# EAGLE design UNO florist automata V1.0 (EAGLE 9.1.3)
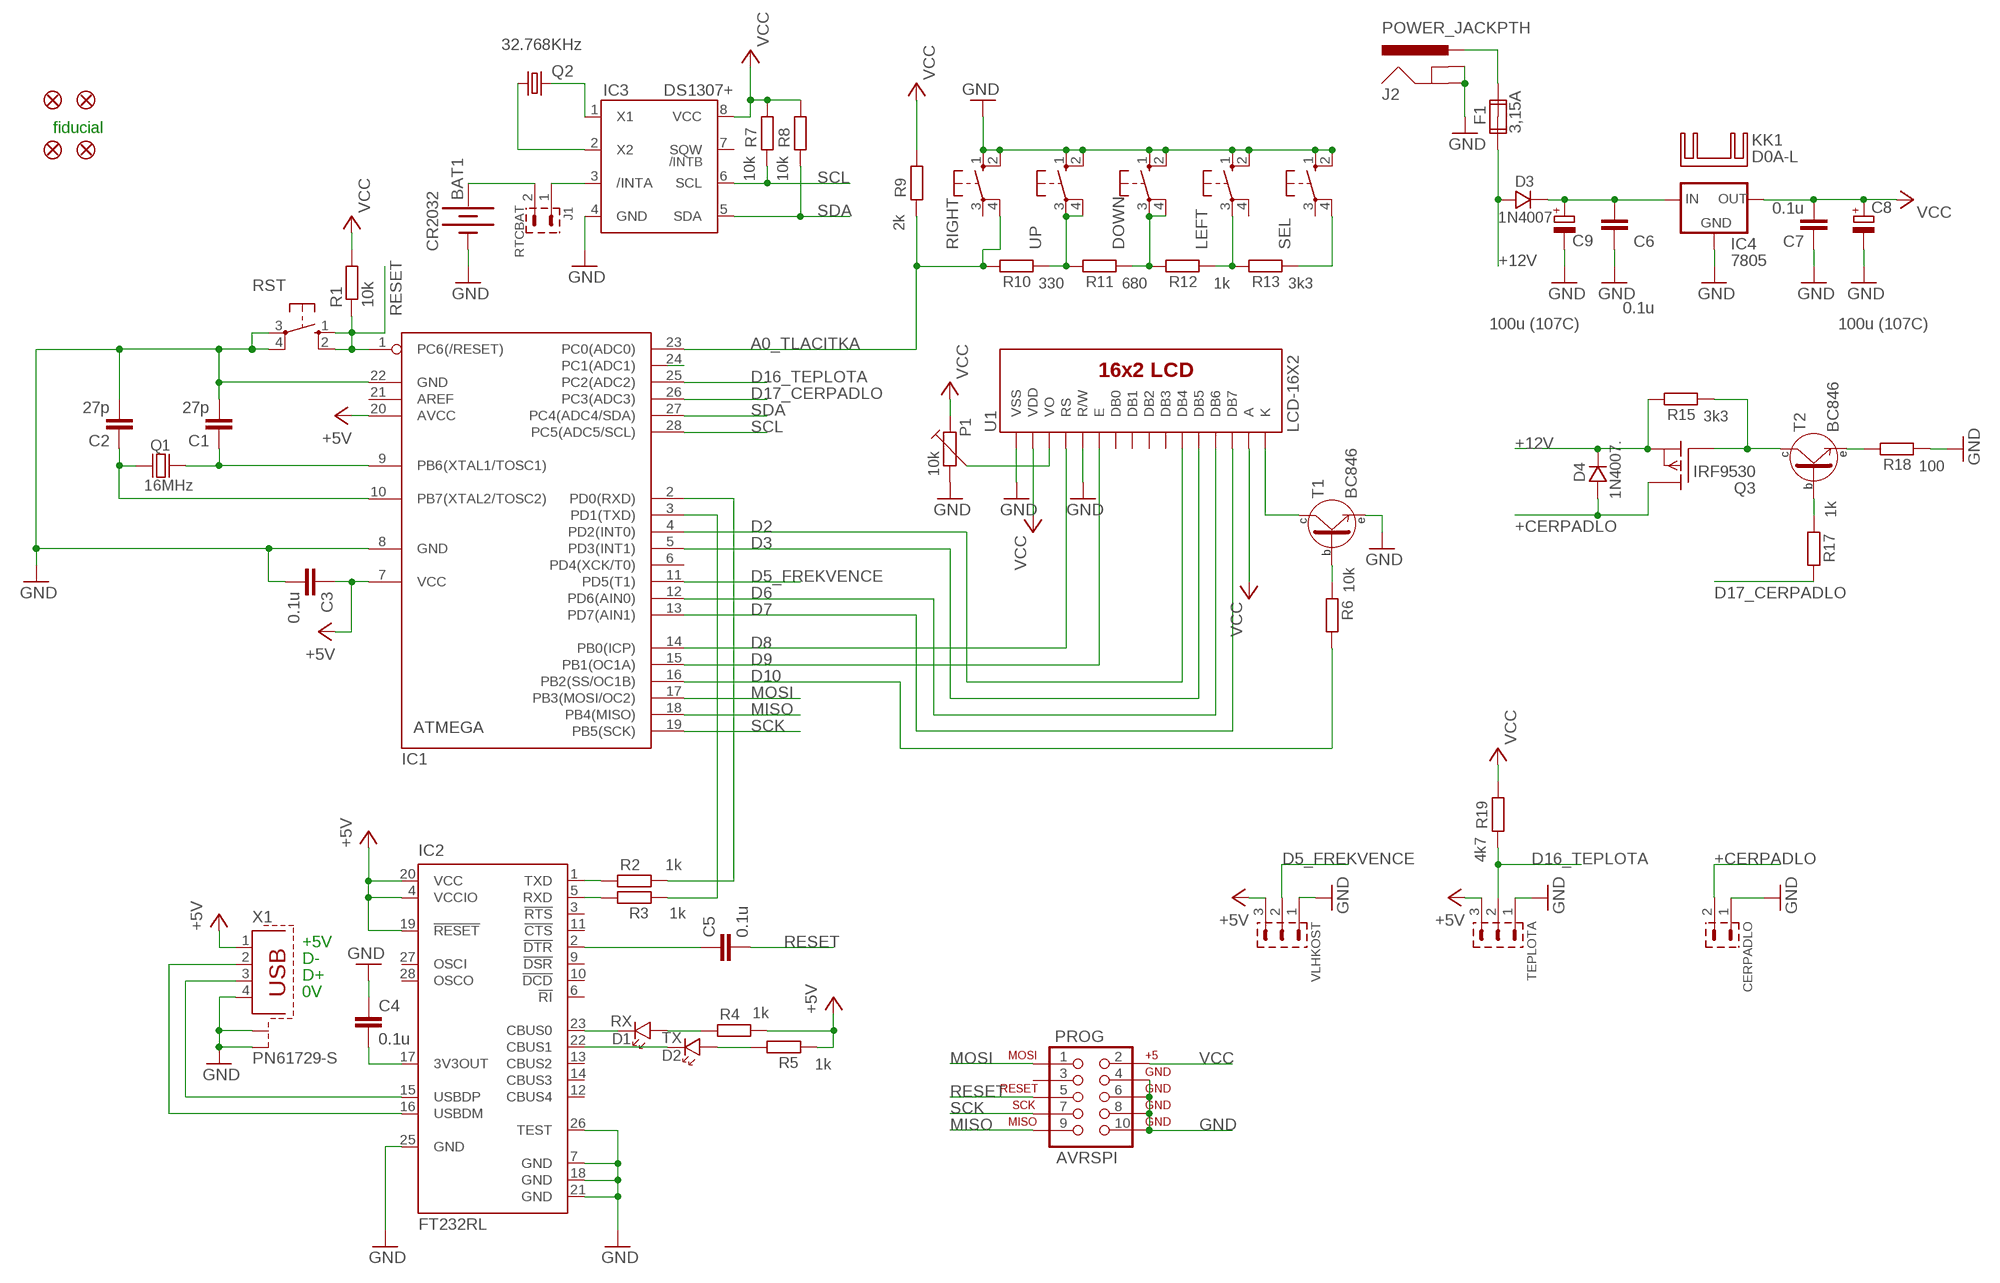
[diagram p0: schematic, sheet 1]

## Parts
BAT1  CR2032  BATTERY20PTH  [BATTCOM_20MM_PTH]
C1  27p  C-EUC1206  [C1206]
C2  27p  C-EUC1206  [C1206]
C3  0.1u  C-EUC1206  [C1206]
C4  0.1u  C-EUC1206  [C1206]
C5  0.1u  C-EUC1206  [C1206]
C6  0.1u  C-EUC1206  [C1206]
C7  0.1u  C-EUC1206  [C1206]
C8  100u (107C)  CPOL-EUC/6032-28W  [C/6032-28W]
C9  100u (107C)  CPOL-EUC/6032-28W  [C/6032-28W]
CERPADLO  PSH02-02P  [PSH02-02P]
D1  RX  LED_1206  [P1206]
D2  TX  LED_1206  [P1206]
D3  1N4007.  [SM-1]
D4  1N4007.  [SM-1]
DOWN  10-XX  [B3F-10XX]
F1  3,15A  FUSE2P  [FUSE1]
FID1  FIDUCIAL1.5X3  [FIDUCIAL-1.5X3]
FID2  FIDUCIAL1.5X3  [FIDUCIAL-1.5X3]
FID3  FIDUCIAL1.5X3  [FIDUCIAL-1.5X3]
FID4  FIDUCIAL1.5X3  [FIDUCIAL-1.5X3]
IC1  ATMEGA  MEGA8-P  [DIL28-3]
IC2  FT232RL  [SSOP28]
IC3  DS1307+  DS1337S+  [SO08]
IC4  7805  78XXL  [78XXL]
J1  RTCBAT  S1G2_JUMP  [S1G2_JUM]
J2  POWER_JACKPTH  [POWER_JACK_PTH]
KK1  D0A-L  [D02A-L]
LEFT  10-XX  [B3F-10XX]
P1  10k  TRIMRPT10V  [PT10V]
PROG  AVRSPI  AVR_SPI_PROG2LOCK  [2X5-SHROUDED_LOCK]
Q1  16MHz  Q_HC-49U  [HC-49U]
Q2  32.768KHz  CRYSTALTC38H  [TC38H]
Q3  IRF9530  [TO220]
R1  10k  R-EU_M1206  [M1206]
R2  1k  R-EU_M1206  [M1206]
R3  1k  R-EU_M1206  [M1206]
R4  1k  R-EU_M1206  [M1206]
R5  1k  R-EU_M1206  [M1206]
R6  10k  R-EU_M1206  [M1206]
R7  10k  R-EU_M1206  [M1206]
R8  10k  R-EU_M1206  [M1206]
R9  2k  R-EU_M1206  [M1206]
R10  330  R-EU_M1206  [M1206]
R11  680  R-EU_M1206  [M1206]
R12  1k  R-EU_M1206  [M1206]
R13  3k3  R-EU_M1206  [M1206]
R15  3k3  R-EU_M1206  [M1206]
R17  1k  R-EU_M1206  [M1206]
R18  100  R-EU_M1206  [M1206]
R19  4k7  R-EU_M1206  [M1206]
RIGHT  10-XX  [B3F-10XX]
RST  10-XX  [B3F-10XX]
SEL  10-XX  [B3F-10XX]
T1  BC846  [SOT-23]
T2  BC846  [SOT-23]
TEPLOTA  PSH02-03P  [PSH02-03P]
U1  LCD-16X2  LCD-16X2NOSILK  [LCD-16X2_NOSILK]
UP  10-XX  [B3F-10XX]
VLHKOST  PSH02-03P  [PSH02-03P]
X1  PN61729-S  [PN61729-S]

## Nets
+12V: D3.A D4.K F1.1A Q3.3(S) R15.2
+CERPADLO: CERPADLO.2 D4.A Q3.2(D)
A: IC3.2(X2) Q2.1
A0_TLACITKA: IC1.23(PC0(ADC0)) R9.1 R10.2 RIGHT.4(P1)
A1_OSVETLENI: IC1.24(PC1(ADC1))
D2: IC1.4(PD2(INT0)) U1.11(DB4)
D3: IC1.5(PD3(INT1)) U1.12(DB5)
D5_FREKVENCE: IC1.11(PD5(T1)) VLHKOST.2
D6: IC1.12(PD6(AIN0)) U1.13(DB6)
D7: IC1.13(PD7(AIN1)) U1.14(DB7)
D8: IC1.14(PB0(ICP)) U1.4(RS)
D9: IC1.15(PB1(OC1A)) U1.6(E)
D10: IC1.16(PB2(SS/OC1B)) R6.2
D16_TEPLOTA: IC1.25(PC2(ADC2)) R19.1 TEPLOTA.2
D17_CERPADLO: IC1.26(PC3(ADC3)) R17.2
GND: BAT1.2(-) C1.2 C2.2 C3.2 C4.1 C6.1 C7.1 C8.- C9.- CERPADLO.1 DOWN.1(S) DOWN.2(S1) IC1.8(GND) IC1.22(GND) IC2.7(GND) IC2.18(GND) IC2.21(GND) IC2.25(GND) IC2.26(TEST) IC3.4(GND) IC4.GND J2.GND J2.GNDBREAK LEFT.1(S) LEFT.2(S1) P1.2 PROG.4 PROG.6 PROG.8 PROG.10 R18.1 RIGHT.1(S) RIGHT.2(S1) RST.3(P) RST.4(P1) SEL.1(S) SEL.2(S1) T1.2(E) TEPLOTA.1 U1.1(VSS) U1.5(R/W) UP.1(S) UP.2(S1) VLHKOST.1 X1.4 X1.S1 X1.S2
MISO: IC1.18(PB4(MISO)) PROG.9
MOSI: IC1.17(PB3(MOSI/OC2)) PROG.1
N$1: IC2.16(USBDM) X1.2
N$2: IC2.15(USBDP) X1.3
N$3: C4.2 IC2.17(3V3OUT)
N$4: IC2.1(TXD) R2.1
N$5: IC2.5(RXD) R3.2
N$6: IC1.2(PD0(RXD)) R2.2
N$7: IC1.3(PD1(TXD)) R3.1
N$8: C5.1 IC2.2(!DTR)
N$9: D1.K IC2.23(CBUS0)
N$10: D1.A R4.1
N$11: D2.K IC2.22(CBUS1)
N$12: D2.A R5.2
N$13: BAT1.1(+) J1.2
N$14: IC3.3(/INTA) J1.1
N$15: T1.3(C) U1.16(K)
N$18: R10.1 R11.2 UP.3(P) UP.4(P1)
N$19: DOWN.3(P) DOWN.4(P1) R11.1 R12.2
N$20: LEFT.3(P) R12.1 R13.2
N$21: R13.1 SEL.4(P1)
N$22: F1.2A J2.PWR
N$23: C1.1 IC1.9(PB6(XTAL1/TOSC1)) Q1.2
N$24: C6.2 C9.+ D3.K IC4.IN
N$25: R6.1 T1.1(B)
N$26: C2.1 IC1.10(PB7(XTAL2/TOSC2)) Q1.1
N$27: Q3.1(G) R15.1 T2.3(C)
N$28: R18.2 T2.2(E)
N$29: R17.1 T2.1(B)
N$31: P1.3 U1.3(VO)
Q1: IC3.1(X1) Q2.2
RESET: C5.2 IC1.1(PC6(/RESET)) PROG.5 R1.1 RST.1(S) RST.2(S1)
SCK: IC1.19(PB5(SCK)) PROG.7
SCL: IC1.28(PC5(ADC5/SCL)) IC3.6(SCL) R7.1
SDA: IC1.27(PC4(ADC4/SDA)) IC3.5(SDA) R8.1
VCC: C3.1 C7.2 C8.+ IC1.7(VCC) IC1.20(AVCC) IC2.4(VCCIO) IC2.19(!RESET) IC2.20(VCC) IC3.8(VCC) IC4.OUT P1.1 PROG.2 R1.2 R4.2 R5.1 R7.2 R8.2 R9.2 R19.2 TEPLOTA.3 U1.2(VDD) U1.15(A) VLHKOST.3 X1.1 ; supply symbol labelled +5V
Unconnected: F1.1B F1.2B IC1.6(PD4(XCK/T0)) IC1.21(AREF) IC2.3(!RTS) IC2.6(!RI) IC2.9(!DSR) IC2.10(!DCD) IC2.11(!CTS) IC2.12(CBUS4) IC2.13(CBUS2) IC2.14(CBUS3) IC2.27(OSCI) IC2.28(OSCO) IC3.7(SQW) LEFT.4(P1) PROG.3 RIGHT.3(P) SEL.3(P) U1.7(DB0) U1.8(DB1) U1.9(DB2) U1.10(DB3)

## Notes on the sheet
- fiducial
- +5V
- D-
- D+
- 0V

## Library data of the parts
BAT1 = SparkFun-Electromechanical:BATTERY: Battery Holders
C1-C7 = rcl:C-EU: CAPACITOR, European symbol
C8 C9 = rcl:CPOL-EU: POLARIZED CAPACITOR, European symbol
CERPADLO = #PaJa_konektory:PSH02-02: Konektory se zamkem - vidlice - 2pin
D1 D2 = #PaJa_31:LED: LED - jednobarevna
D3 D4 = #PaJa_31:1N4007: Usmernovaci dioda - 1A, 1000V
DOWN LEFT RIGHT RST SEL UP = switch-omron-modified:10-XX: OMRON SWITCH
F1 = special:FUSE2P: FUSE 5 x 20 mm
FID1-FID4 = SparkFun-Retired:FIDUCIAL: Fiducial Alignment Points
IC1 = atmel:MEGA8-P: MICROCONTROLLER 8 Kbytes FLASH, 1 kbytes SRAM, 512 bytes EEPROM, USART, 4-channel 10 bit ADC, 2-channel 8 bit ADC Pin compatible with Atmega48, ATMega88, ATMega168 Source: avr.lbr
IC2 = ftdichip:FT232R: Source: http://www.ftdichip.com/Documents/DataSheets/DS_FT232R_v104.pdf; MPN: FT232RL; OC_FARNELL: 1146032; OC_NEWARK: 91K9918
IC3 = #PaJa_31:DS1337: RTC - obvod realneho casu (ekviv. DS1307)
IC4 = v-reg:78XXL: VOLTAGE REGULATOR
J1 = #PaJa_konektory:S1G2_JUMP: Radove konektory - koliky - 2x
J2 = SparkFun-Connectors:POWER_JACK: Power Jack This is the standard 5.5mm barrel jack for power. The PTH is the most common, proven, reliable, footprint. The Slot footprint only works if the mill layer is transmitted to the PCB fab house so be warned. Mating wall wart : TOL-00298 (and others); PROD_ID: PRT-00119
KK1 = heatsink:D0A-L: HEATSINK
P1 = #PaJa_31:TRIMR: Trimr
PROG = SparkFun-Connectors:AVR_SPI_PROG2: AVR 10-pin ICSP Header This is the standard AVR In Circuit Serial Programming header. Minimal, but includes pin one indicator. Works with standard Olimex programmers. Also look for the 6-pin reduced version. Spark Fun Electronics SKU: PRT-00778
Q1 = #PaJa_31:Q: Krystal
Q2 = crystal:CRYSTAL: CRYSTAL; OC_FARNELL: unknown; OC_NEWARK: unknown
Q3 = transistor-fet:IRF9530: P-Channel Enhancement MOSFET (HEXFET); -100V; -12A; 0,3Ohm
R1-R13 R15 R17-R19 = rcl:R-EU_: RESISTOR, European symbol
T1 T2 = #PaJa_31:BC846: SMD tranzistor - NPN - ekv. BC546
TEPLOTA VLHKOST = #PaJa_konektory:PSH02-03: Konektory se zamkem - vidlice - 3pin
U1 = SparkFun-Displays:LCD-16X2: Standard text-only 16x2 parallel input LCD
X1 = con-berg:PN61729-S: BERG USB connector; OC_FARNELL: unknown; OC_NEWARK: unknown

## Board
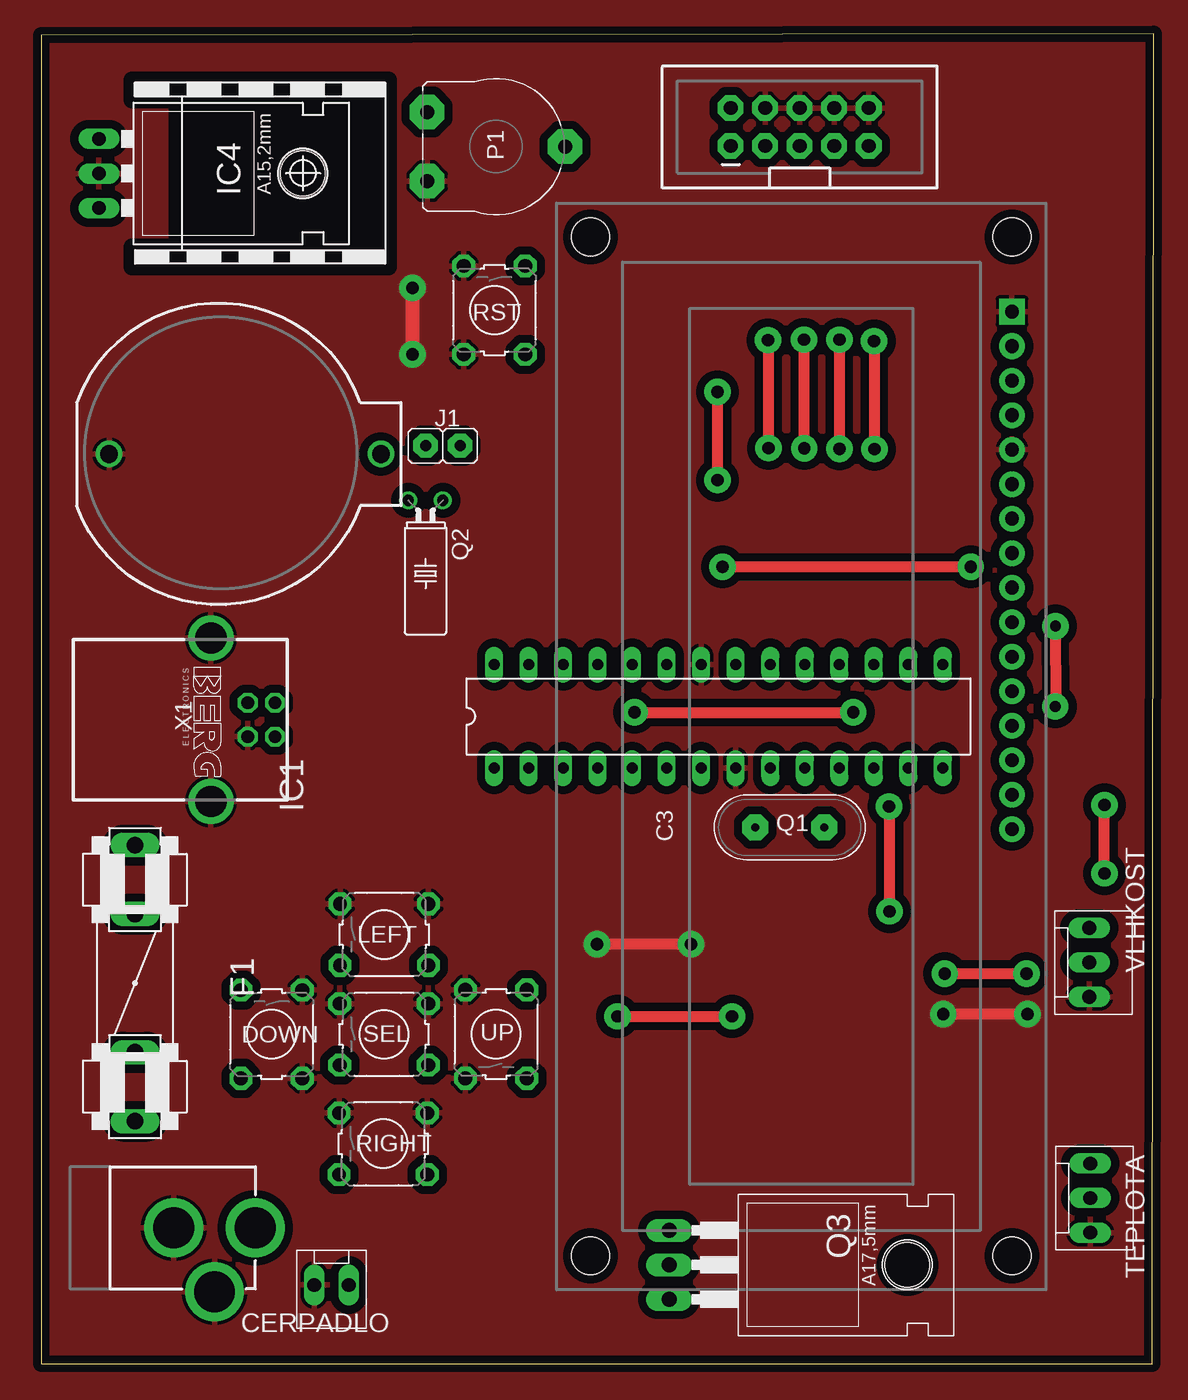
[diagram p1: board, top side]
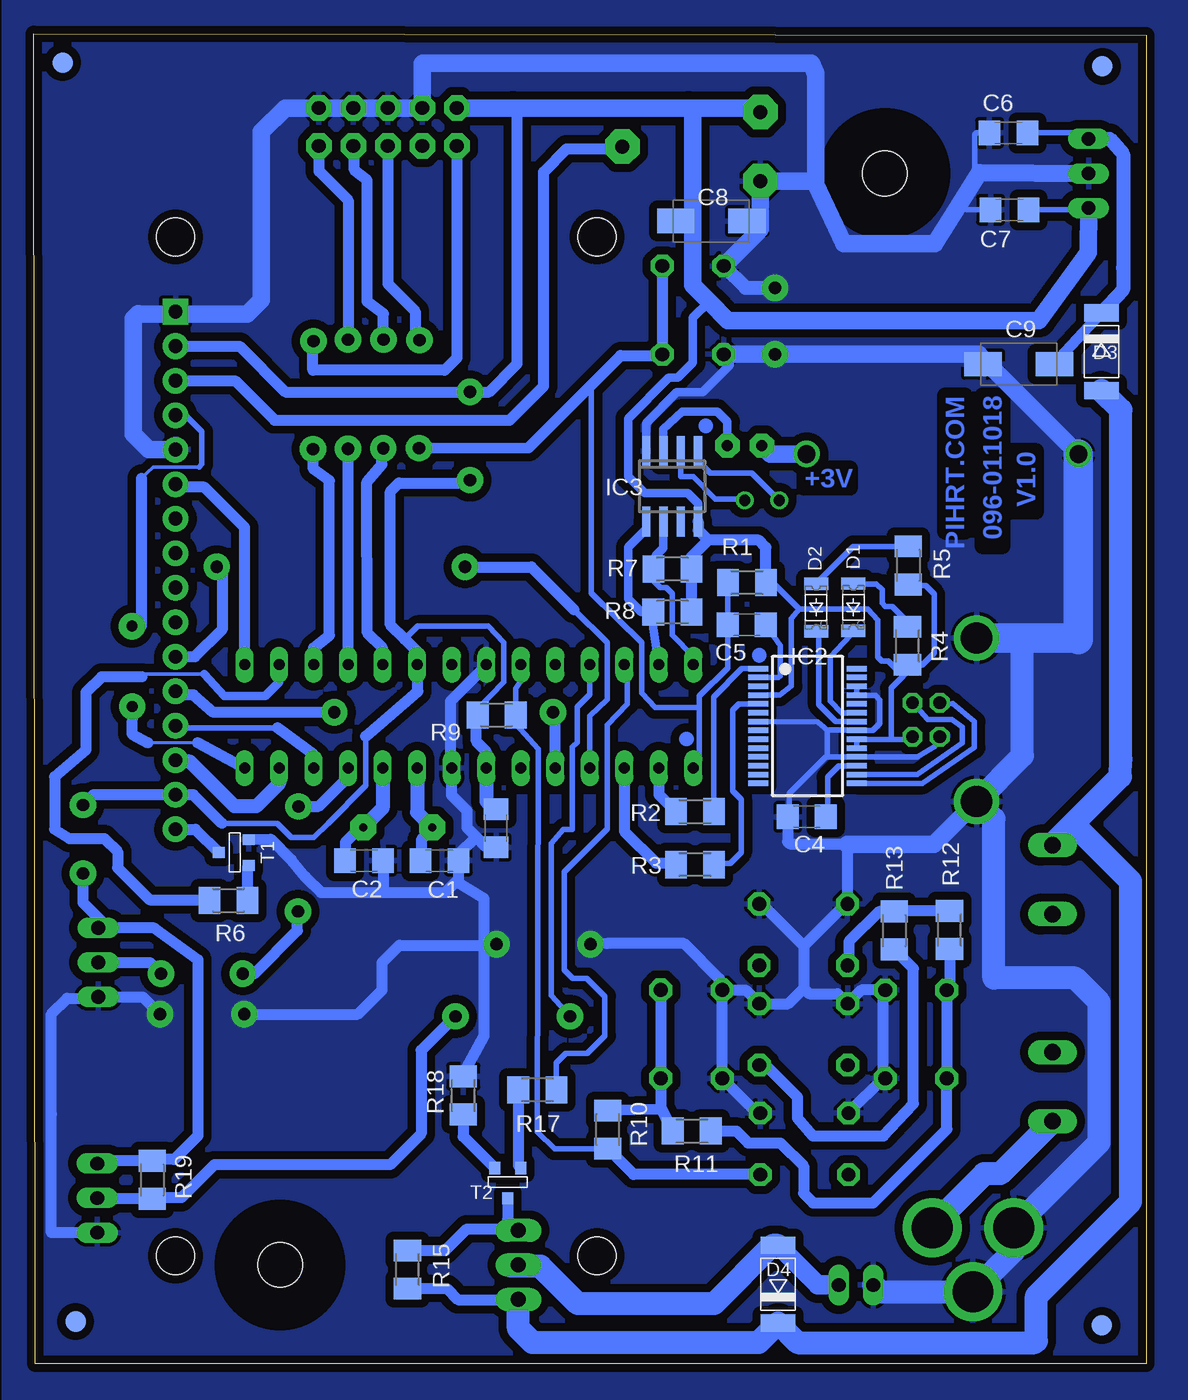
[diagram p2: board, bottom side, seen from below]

Size 81.85 x 97.9 mm. Coordinates in mm from the lower left corner, seen from the top.
Outline: 0.02,0.01 81.76,0 81.85,97.9 0,97.8 0.02,0.01
Copper layers (1*16): Top 0.035mm / dielectric 1.5mm / Bottom 0.035mm
Design rules "default": minimum track width 5mil, minimum drill 12mil, track to track 5mil, track to pad 5mil, pad to pad 5mil, via to via 5mil, smd to smd 0mil, copper to edge 10mil, drill to drill 10mil, minimum pad ring 10mil, minimum via ring 6mil, stop-mask expansion 2mil, vias tented up to drill 25mil, thermal gap 10mil

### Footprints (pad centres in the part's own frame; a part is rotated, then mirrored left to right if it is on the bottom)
BATTCOM_20MM_PTH = drill 1.3: 1 11.85,0; 2 -8.15,0
C1206 = smd 1.6 x 1.8: 1 -1.4,0; 2 1.4,0
C/6032-28W = smd 2.75 x 1.8: + 2.625,0; - -2.625,0
PSH02-02P = drill 1.016 pad 1.422 long: 1 -1.27,0; 2 1.27,0
P1206 = smd 0.914 x 1.778: A -1.905,0; K 1.587,0
SM-1 = smd 1.27 x 2.54: A 2.857,0; K -2.857,0
B3F-10XX = drill 1.016 pad 1.676 octagon: 1 -3.251,2.261; 2 3.251,2.261; 3 -3.251,-2.261; 4 3.251,-2.261
FUSE1 = drill 1.194 long: 1A -10.16,0; 1B -5.08,0; 2A 10.16,0; 2B 5.08,0
FIDUCIAL-1.5X3 = smd 1.5 x 1.5: 1 0,0
DIL28-3 = drill 0.813 long: 1 -16.51,-3.81; 2 -13.97,-3.81; 3 -11.43,-3.81; 4 -8.89,-3.81; 5 -6.35,-3.81; 6 -3.81,-3.81; 7 -1.27,-3.81; 8 1.27,-3.81; 9 3.81,-3.81; 10 6.35,-3.81; 11 8.89,-3.81; 12 11.43,-3.81; 13 13.97,-3.81; 14 16.51,-3.81; 15 16.51,3.81; 16 13.97,3.81; 17 11.43,3.81; 18 8.89,3.81; 19 6.35,3.81; 20 3.81,3.81; 21 1.27,3.81; 22 -1.27,3.81; 23 -3.81,3.81; 24 -6.35,3.81; 25 -8.89,3.81; 26 -11.43,3.81; 27 -13.97,3.81; 28 -16.51,3.81
SSOP28 = smd 0.4 x 1.5: 1 -4.225,-3.625; 2 -3.575,-3.625; 3 -2.925,-3.625; 4 -2.275,-3.625; 5 -1.625,-3.625; 6 -0.975,-3.625; 7 -0.325,-3.625; 8 0.325,-3.625; 9 0.975,-3.625; 10 1.625,-3.625; 11 2.275,-3.625; 12 2.925,-3.625; 13 3.575,-3.625; 14 4.225,-3.625; 15 4.225,3.625; 16 3.575,3.625; 17 2.925,3.625; 18 2.275,3.625; 19 1.625,3.625; 20 0.975,3.625; 21 0.325,3.625; 22 -0.325,3.625; 23 -0.975,3.625; 24 -1.625,3.625; 25 -2.275,3.625; 26 -2.925,3.625; 27 -3.575,3.625; 28 -4.225,3.625
SO08 = smd 0.6 x 2.2: 1 -1.905,-2.6; 2 -0.635,-2.6; 3 0.635,-2.6; 4 1.905,-2.6; 5 1.905,2.6; 6 0.635,2.6; 7 -0.635,2.6; 8 -1.905,2.6
78XXL = drill 1.016 long: GND 0,-3.81; IN -2.54,-3.81; OUT 2.54,-3.81 | hole 3.302: 0,11.176
S1G2_JUM = drill 0.813 pad 1.778 octagon: 1 -1.27,0; 2 1.27,0
POWER_JACK_PTH = drill 2.997 pad 4.318: GND 0,7.7; GNDBREAK 4.7,10.7; PWR 0,13.7
PT10V = drill 1.016 pad 2.54 octagon: 1 -2.54,-5.08; 2 2.54,-5.08; 3 0,5.08
2X5-SHROUDED_LOCK = drill 1.016 pad 1.88 octagon: 1 -1.397,5.08; 2 1.397,5.08; 3 -1.397,2.54; 4 1.397,2.54; 5 -1.397,0; 6 1.397,0; 7 -1.397,-2.54; 8 1.397,-2.54; 9 -1.397,-5.08; 10 1.397,-5.08
HC-49U = drill 0.61 pad 1.93 octagon: 1 -2.54,0; 2 2.54,0
TC38H = drill 0.813: 1 -1.27,0; 2 1.27,0
TO220 = drill 1.118 long: 1 -2.54,-6.35; 2 0,-6.35; 3 2.54,-6.35 | hole 3.302: 0,11.176
M1206 = smd 1.6 x 2: 1 -1.4,0; 2 1.4,0
SOT-23 = smd 0.787 x 0.889: 1 -0.953,-0.953; 2 0.953,-0.953; 3 0,1.27
PSH02-03P = drill 1.016 pad 1.422 long: 1 -2.54,0; 2 0,0; 3 2.54,0
LCD-16X2_NOSILK = drill 1.016 pad 1.88 square: 1 -32,15.5 | drill 1.016 pad 1.88: 2 -29.46,15.5; 3 -26.92,15.5; 4 -24.38,15.5; 5 -21.84,15.5; 6 -19.3,15.5; 7 -16.76,15.5; 8 -14.22,15.5; 9 -11.68,15.5; 10 -9.14,15.5; 11 -6.6,15.5; 12 -4.06,15.5; 13 -1.52,15.5; 14 1.02,15.5; 15 3.56,15.5; 16 6.1,15.5 | hole 2.8: -37.5,15.5; -37.5,-15.5; 37.5,15.5; 37.5,-15.5
PN61729-S = drill 0.95 octagon: 1 1.25,4.71; 2 -1.25,4.71; 3 -1.25,2.71; 4 1.25,2.71 | drill 2.3 pad 2.9: S1 -6.02,0; S2 6.02,0

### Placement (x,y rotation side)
BAT1  13.16,66.97 0 top
C1  52.02,37.05 0 bottom
C2  57.57,37.05 0 bottom
C3  47.86,39.43 270 bottom
C4  25,40.27 0 bottom
C5  29.41,54.41 180 bottom
C6  10.15,90.61 0 bottom
C7  10.07,84.95 0 bottom
C8  32.01,84.13 180 bottom
C9  9.4,73.59 0 bottom
CERPADLO  21.37,5.81 0 top
D1  21.56,55.54 270 bottom
D2  24.3,55.53 270 bottom
D3  3.3,74.51 270 bottom
D4  27.09,5.87 90 bottom
DOWN  16.96,24.27 270 top
F1  6.9,28.03 270 top
FID1  3.24,95.51 0 bottom
FID2  3.28,2.84 0 bottom
FID3  79.75,95.8 0 bottom
FID4  78.79,3.12 0 bottom
IC1  49.84,47.67 0 top
IC2  24.94,46.96 270 bottom
IC3  34.9,64.61 180 bottom
IC4  8.07,87.63 270 top
J1  29.56,67.59 180 top
J2  2.06,10.02 270 top
KK1  13.81,87.64 180 top
LEFT  25.25,31.61 0 top
P1  33.48,89.6 270 top
PROG  55.82,91.05 90 top
Q1  55.08,39.5 180 top
Q2  28.29,63.57 180 top
Q3  52.56,7.3 270 top
R1  29.39,57.51 0 bottom
R2  33.22,40.66 180 bottom
R3  33.22,36.74 0 bottom
R4  17.58,52.86 270 bottom
R5  17.52,58.78 90 bottom
R6  67.54,34.13 180 bottom
R7  34.87,58.52 0 bottom
R8  34.88,55.34 0 bottom
R9  47.81,47.76 180 bottom
R10  39.63,17.26 270 bottom
R11  33.45,17.15 180 bottom
R12  14.49,31.94 270 bottom
R13  18.55,31.91 90 bottom
R15  54.37,6.95 270 bottom
R17  44.81,20.18 0 bottom
R18  50.27,19.77 270 bottom
R19  73.15,13.55 90 bottom
RIGHT  25.17,16.21 0 top
RST  33.36,77.57 270 top
SEL  25.23,24.26 0 top
T1  66.99,37.65 90 bottom
T2  46.99,13.47 180 bottom
TEPLOTA  77.19,12.21 90 top
U1  55.94,45.46 270 top
UP  33.48,24.28 90 top
VLHKOST  77.13,29.55 90 top
X1  12.5,47.42 270 top

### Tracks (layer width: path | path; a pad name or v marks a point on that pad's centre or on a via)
+12V
  Bottom 0.813: R15.2 51.48,5.55 50.65,4.73 46.24,4.73 Q3.3
  Bottom 1.676: D3.A 1.88,70.23 1.88,44.51 1.92,43.24 5.56,39.6 | 5.56,39.6 6.9,38.26 F1.1A | Q3.3 46.21,2.61 45.15,1.56 28.55,1.56 D4.K 25.64,1.56 8.23,1.56 8.09,1.69 8.09,5 1.15,11.94 1.15,35.52 5.23,39.6 5.56,39.6
+CERPADLO
  Bottom 1.422: CERPADLO.2 24.18,5.81 D4.A
  Bottom 1.676: D4.A 27.52,8.73 31.81,4.44 41.84,4.44 44.59,7.2 46.75,7.2 46.8,7.25 46.25,7.25 Q3.2
A
  Bottom 0.406: Q2.1 29.66,63.67 31.72,63.67 33.35,65.3 34.27,65.3 IC3.2
A0_TLACITKA
  Bottom 0.406: IC1.23 45.84,51.29 45.84,50.53 46.41,49.7 R9.1 46.41,47.12 44.77,45.26 44.81,17.1 43.54,15.83 39.66,15.83 R10.2
  Bottom 0.813: R10.2 37.72,13.94 RIGHT.4
D2  (via drill 0.9 pad 1.93)
  Top 0.813: v68.4,58.67 v50.14,58.67
  Bottom 0.406: IC1.4 40.95,47.68 39.67,48.92 39.67,53.12 42.12,55.53
  Bottom 0.813: U1.11 70.02,52.06 67.97,54.1 67.97,58.24 v68.4,58.67 | v50.14,58.67 45.26,58.67 42.12,55.53
D3  (via drill 0.9 pad 1.93)
  Top 0.813: v43.66,47.97 v59.76,47.97
  Bottom 0.813: IC1.5 43.49,47.64 v43.66,47.97 | v59.76,47.97 68.65,47.97 70.12,49.25 71.17,49.25 U1.12
D5_FREKVENCE  (via drill 0.9 pad 1.93)
  Top 0.813: v72.5,28.73 v66.5,28.73 | v62.43,33.31 62.43,41 v62.39,41.04
  Bottom 0.813: VLHKOST.2 73.33,29.55 v72.5,28.73 | v66.5,28.73 65.64,28.73 62.47,31.9 62.47,33.28 v62.43,33.31 | v62.39,41.04 60.9,41.04 58.89,43.05 58.89,43.7 IC1.11
D6
  Bottom 0.406: IC1.12 61.27,44.85 | 63.92,46.83 71.04,46.83 U1.13
  Bottom 0.813: 61.27,44.85 63.92,46.83
D7
  Bottom 1.016: IC1.13 63.81,42.74 65.5,41.05 67.09,41.05 70.37,44.34 71.34,44.34 U1.14
D8  (via drill 0.8 pad 1.93)
  Top 0.813: v74.64,54.3 74.65,48.55 v74.63,48.39
  Bottom 0.254: 69.67,66.03 73.09,66.03 73.95,65.19 | 73.45,45.71 69.82,45.73
  Bottom 0.406: U1.4 70.71,69.84 69.5,68.63 69.5,66.23 69.67,66.03
  Bottom 0.813: 73.95,65.19 73.95,54.34 v74.64,54.3 | v74.63,48.39 74.64,46.37 73.45,45.71 | 69.82,45.73 IC1.14
D9
  Bottom 0.813: IC1.15 66.35,61.58 69.31,64.54 71.22,64.54 U1.6
D10
  Bottom 0.254: 69.31,50.8 73.92,50.8 73.9,50.58
  Bottom 0.61: IC1.16 63.81,50.19 64.84,49.16 67.84,49.16 69.31,50.8
  Bottom 0.813: 73.9,50.58 76.88,50.58 78.03,49.43 78.03,45.2 80.33,43.24 80.33,39.36 79.24,38.67 76.66,38.67 75.7,37.71 75.7,36.53 73.34,34.17 68.97,34.17 R6.2
D16_TEPLOTA  (via drill 0.9 pad 1.93)
  Top 0.813: v42.41,25.59 v50.83,25.59
  Bottom 0.406: IC1.25 40.95,49.26 41.86,48.35 41.86,45.76 42.23,45.41 42.23,39.35 42.89,39.35 43.81,38.31 43.81,27.12 v42.41,25.59
  Bottom 0.813: TEPLOTA.2 77.13,12.15 R19.1 73.06,12.24 71.01,12.24 68.59,14.66 55.64,14.66 53.37,16.94 53.37,23.09 50.87,25.59 v50.83,25.59
D17_CERPADLO
  Bottom 0.406: IC1.26 38.19,51.26 38.19,48.57 39.68,47.02 39.68,39.37 42.84,36.21 42.84,29.02 42.22,28.39 41.18,28.39 39.85,27.06 39.85,24.17 41.14,22.88 42.71,22.88 43.41,22.17 R17.2
GND  (via drill 0.9 pad 1.93)
  Top 0.813: v40.91,30.9 v47.82,30.9 | v72.58,25.74 v66.39,25.74
  Top 1.016: v27.32,79.21 v27.32,74.32
  Bottom 0.406: IC2.26 IC2.25 21.27,49.21 19.92,49.21 19.62,48.88 19.62,47.13 20.12,46.64 IC2.21 21.33,46.65 | X1.4 15.58,45.44 16.85,44.67 20.99,44.67 IC2.18 23.58,44.68 | IC2.7 24.18,47.27 23.45,46.63 21.33,46.65 | 23.58,44.68 26.28,41.98 26.28,40.24 26.28,40.07 26.4,40.07 | 21.33,46.65 23.46,46.65 23.5,46.61 23.5,44.77 23.58,44.68 | C6.1 12.5,90.61 12.64,90.47 12.64,88.04 12.29,87.69 | C7.1 13.2,84.95 13.7,85.44
  Bottom 0.61: IC3.4 36.8,69.27 34.54,71.53 32.65,71.53 30.65,73.53 30.65,73.87 RST.4
  Bottom 0.813: C3.2 48.56,38.03 49.33,38.8 | 49.33,38.8 49.98,39.45 49.98,40.72 51.12,41.86 IC1.8 51.21,43.95 51.21,48.77 48.57,51.4 IC1.22 | 49.33,38.8 50.62,37.51 C1.2 50.6,37.03 50.6,35.68 50.77,35.51 | C4.1 26.31,40.27 26.28,40.24 | 26.4,40.07 26.4,38.43 26.26,38.28 22.07,38.28 22.03,38.25 22.03,33.9 LEFT.1 22.14,33.87 25.23,30.78 | T1.2 64.43,38.63 62.91,37.11 61.89,35.86 60.73,34.7 56.04,34.7 | 56.04,34.7 51.58,34.7 50.77,35.51 | C2.2 56.17,34.83 56.04,34.7 | DOWN.2 19.37,21.02 | 19.37,21.02 RIGHT.1 | RIGHT.2 28.66,18.47 UP.1 | 25.23,30.78 25.23,27.66 | 25.23,27.66 24.82,27.25 22.71,27.25 SEL.1 20.97,27.52 DOWN.1 19.37,27.37 19.37,21.02 | 25.23,27.66 26.36,26.52 SEL.2 29.49,27.53 UP.2 UP.1 | LEFT.2 28.31,33.87 25.23,30.78 | 71.63,77.26 U1.1 | UP.1 31.22,27.57 31.41,27.76 31.41,28.35 34.01,30.94 39.7,30.94 v40.91,30.9 | R18.1 50.27,21.3 48.73,24.14 48.73,30.67 | 48.73,30.67 48.73,30.86 | 48.73,30.86 v47.82,30.9 | 48.73,30.86 48.73,34.25 50.77,35.51 | TEPLOTA.1 80.57,9.67 80.58,9.67 80.58,18.41 80.58,25.75 79.41,26.91 77.22,26.91 VLHKOST.1 73.84,27.01 v72.58,25.74 | v66.39,25.74 58.03,25.74 56.24,27.53 56.24,29.55 54.97,30.81 48.88,30.81 48.73,30.67 | C9.- 12.21,74.18 | C8.- 28.68,83.24
  Bottom 1.016: RST.3 29.48,79.21 v27.32,79.21
  Bottom 1.27: RST.3 28.68,83.24 28.4,83.51 P1.2 28.39,87.08 24.6,87.06 | IC4.GND 12.29,87.69 13.7,85.44 15.55,82.47 22.25,82.47 24.36,86.89 24.6,87.06 | 24.6,87.06 24.32,87.13 24.32,94.98 24.67,95.74 53.26,95.74 53.28,95.72 PROG.4 PROG.6 PROG.8 PROG.10 63.37,92.45 65.12,90.7 65.12,78.3 66.15,77.26 71.63,77.26 74.13,77.26 74.17,77.3 74.54,76.92 74.54,68.43 73.41,67.3 U1.5 | RST.4 v27.32,74.32 12.35,74.32 12.21,74.18 BAT1.2 | X1.S2 15.65,38.25 22.03,38.25
  Bottom 1.676: CERPADLO.1 19.6,5.31 J2.GNDBREAK 9.76,8.31 J2.GND 3.47,16.3 3.47,26.63 5.25,28.41 11.22,28.41 11.22,40.12 X1.S2 9.13,44.77 9.13,53.44
  Bottom 2.184: BAT1.2 5.01,53.31 5.14,53.44 9.13,53.44 X1.S1
  pour Bottom (isolate 0.61): -4.02,100.89 -4.02,-2.8 84.05,-2.8 84.05,100.89
  pour Top (isolate 0.61): -4.28,101.93 -4.28,-3.54 85.41,-3.54 85.41,101.93
MISO  (via drill 0.9 pad 1.93)
  Top 0.813: v58.74,75.39 v58.74,67.36
  Bottom 0.813: PROG.9 60.86,89.62 60.86,87.78 58.74,85.66 v58.74,75.39 | IC1.18 v58.73,67.35 v58.74,67.36
MOSI  (via drill 0.9 pad 1.93)
  Top 0.813: v61.29,75.29 61.29,67.38 v61.32,67.35
  Bottom 0.813: IC1.17 61.27,52.7 60.12,53.63 60.12,65.01 61.3,65.89 v61.32,67.35 | PROG.1 50.74,74.04 51.64,73.14 61.32,73.14 61.32,74.92 61.31,74.93 61.31,75.27 v61.29,75.29
N$1
  Bottom 0.406: IC2.16 16.85,43.38 13.55,45.7 13.54,46.88 14.34,47.42 16.09,47.43 X1.2
N$2
  Bottom 0.406: IC2.15 16.48,42.73 12.66,45.36 12.66,47.28 14.24,48.63 15.16,48.59 X1.3
N$3
  Bottom 0.406: IC2.17 22.64,44.03 23.46,43.2 23.46,40.34 23.54,40.2
  Bottom 0.813: C4.2 23.54,40.2
N$4
  Bottom 0.406: R2.1 31.82,49.11 29.76,51.19 28.6,51.19 IC2.1
N$5
  Bottom 0.406: IC2.5 29.99,48.58 30.45,48.12 30.45,42.19 29.82,41.56 29.82,37.65 30.64,36.83 31.73,36.83 R3.2
N$6
  Bottom 0.813: IC1.2 35.87,41.91 R2.2
N$7
  Bottom 0.813: IC1.3 38.41,39.2 36.08,36.86 34.74,36.86 R3.1
N$8
  Bottom 0.406: IC2.2 27.09,50.53 26.93,50.65 26.93,52.89 C5.1
N$9
  Bottom 0.406: IC2.23 22.41,47.93 23.26,48.78 23.26,52.05 21.29,54.16 21.06,54.16 D1.K
N$10
  Bottom 0.406: R4.1 17.58,54.64 18.7,55.76 19.2,55.76 19.45,56.01 19.45,57 19.86,57.41 20.77,57.41 D1.A
N$11
  Bottom 0.406: IC2.22 22.85,47.28 24.09,48.53 24.09,54.09 D2.K
N$12
  Bottom 0.406: R5.2 21.56,60.18 D2.A
N$13
  Bottom 1.27: BAT1.1 27.67,66.97 J1.2
N$14
  Bottom 0.61: J1.1 30.83,69.36 31.58,70.11 34.16,70.11 35.53,68.81 35.53,67.27 IC3.3
N$15
  Bottom 0.813: U1.16 69.98,39.36 T1.3
N$18
  Bottom 0.813: UP.4 UP.3 35.73,18.84 R11.2 35.67,18.72 R10.1
N$19
  Bottom 0.813: R12.2 14.49,27.73 DOWN.3 DOWN.4 14.68,21 14.68,17.27 20.1,11.86 24.51,11.86 25.22,12.56 25.22,14.57 26.93,16.27 29.3,16.27 30.18,17.15 R11.1
N$20
  Bottom 0.813: R12.1 18.52,33.34 R13.2 19.67,33.31 21.89,31.09 21.89,29.45 LEFT.3
N$21
  Bottom 0.813: SEL.4 28.04,22 25.69,19.64 25.69,18.1 24.54,16.78 19.35,16.78 17.15,19.15 17.15,29.11 R13.1
N$22
  Bottom 1.676: F1.2A 10.77,14 11.94,14 15.76,10.18 J2.PWR
N$23
  Bottom 0.813: Q1.2 52.54,39.41 53.35,38.59 53.35,37.11 C1.1
  Bottom 1.016: IC1.9 53.65,40.61 Q1.2
N$24
  Bottom 0.406: C6.2 4.7,90.61 IC4.IN
  Bottom 0.813: C9.+ D3.K
  Bottom 1.016: IC4.IN 2.71,90.17 1.71,89.04 1.71,80.69 1.71,79.09 D3.K
N$25
  Bottom 0.813: R6.1 66.14,36.6 T1.1
N$26
  Bottom 0.813: Q1.1 57.84,39.5 58.94,38.4 58.94,37.08 C2.1
  Bottom 1.016: IC1.10 56.19,40.92 Q1.1
N$27
  Bottom 0.813: T2.3 46.99,10.62 Q3.1 46.31,9.94 50,9.94 51.59,8.35 R15.1
N$28
  Bottom 0.813: R18.2 50.27,16.74 T2.2
N$29
  Bottom 0.813: R17.1 46.21,14.59 T2.1
N$31
  Bottom 0.813: U1.3 67.05,72.38 64.14,69.47 46.86,69.47 44.36,71.97 44.36,87.74 42.66,89.44 38.73,89.44 P1.3
Q1
  Bottom 0.406: Q2.2 29.02,65.57 32.1,65.57 32.99,66.45 33.02,66.45 33.02,67.18 IC3.1
RESET  (via drill 0.9 pad 1.93)
  Top 0.813: v53.49,75.36 53.49,67.42 v53.53,67.42
  Bottom 0.406: R1.1 30.79,54.43 C5.2 30.81,51.24 32.89,49.16 32.89,48.2 | 32.89,48.2 32.89,44.3 IC1.1 | 35.72,74.22 38.65,74.22 38.71,74.15 38.8,74.15 40.86,72.09 40.86,56.75 37.14,53.11 37.14,49.39 36.15,48.31 33,48.31 32.89,48.2
  Bottom 0.813: PROG.5 55.82,79.5 53.81,77.49 53.81,75.47 v53.49,75.36 | v53.53,67.42 45.45,67.44 38.69,74.22 35.72,74.22 RST.2 RST.1
SCK  (via drill 0.9 pad 1.93)
  Top 0.813: v56.15,67.39 56.15,74.65 v56.14,75.39
  Bottom 0.813: IC1.19 56.19,52.68 57.33,53.82 57.35,64.92 56.26,66.21 56.26,67.29 v56.15,67.39 | v56.14,75.39 56.14,77.3 57.34,78.21 57.34,87.13 58.28,87.89 58.28,89.58 PROG.7
SCL
  Bottom 0.406: IC1.28 33.33,52.09 34.88,53.64 34.88,56.7 35.34,57.15 35.76,57.15 36.39,57.79 36.39,58.41 R7.1
  Bottom 0.61: IC3.6 35.53,60.06 36.1,59.49 36.1,58.7 R7.1
SDA
  Bottom 0.61: IC3.5 36.8,61.45 38.12,60.13 38.12,56.3 37.16,55.34 R8.1 36.28,54.15 IC1.27
VCC  (via drill 0.9 pad 1.93)
  Top 0.813: v49.77,65.06 v49.77,71.55 | v78.24,36.1 v78.24,41.15
  Bottom 0.406: 18.83,45.98 IC2.20 IC2.19 | 18.83,45.98 17.4,45.98 X1.1 | 17.89,50.64 17.58,50.95 R4.2 16.49,51.46 15.62,52.33 15.62,56.66 16.25,57.28 17.43,57.28 R5.1 | 17.89,50.64 18.78,49.75 18.78,46.03 18.83,45.98 | IC2.4 26.98,49.23 26.13,49.89 26.13,54.87 25.55,55.58 | 25.55,55.58 20.5,55.58 19.75,54.74 19.75,52.04 19.47,51.76 19,51.76 17.89,50.64 | R1.2 27.48,57.51 25.55,55.58 | 57.44,46.19 57.44,42.59 60.2,39.8 61.25,38.75 62.91,38.75 63.97,39.8 68.03,39.8 | 53.6,51.04 IC1.20 53.43,51.7 | C7.2 4.4,84.95 IC4.OUT | R9.2 49.21,48.2 47.3,50.19 47.3,53.09 48.44,54.31 53.62,54.31 54.58,53.35
  Bottom 0.61: IC3.8 32.99,63.33 33.75,64.09 36.91,64.09 38.13,65.31 38.13,69.6 35.13,72.59 34.47,72.59 33.36,73.69 33.36,77 32.17,78.19
  Bottom 0.813: R1.2 27.99,60.1 28.52,60.63 32.26,60.63 | 32.26,60.63 33.49,59.39 33.49,58.54 R7.2 R8.2 | IC3.8 32.99,61.36 32.26,60.63 | 68.03,39.8 70.13,41.9 U1.15 77.49,41.9 v78.24,41.15 | 57.44,46.19 53.6,49.51 53.6,51.04 | U1.2 66.71,74.92 63.35,71.55 v49.77,71.55 48.37,71.55 46.3,73.62 46.3,92.12 46.62,92.45 | IC1.7 48.54,43.89 48.54,45.04 49.3,45.84 49.31,47.66 R9.2 | 53.43,51.7 53.43,52.2 54.58,53.35 55.64,54.41 55.64,64.21 55.01,64.84 50,64.84 v49.77,65.06 | TEPLOTA.3 76.99,14.95 R19.2 73.05,15.05 71.53,15.05 69.79,16.79 69.79,22.21 69.79,23.42 69.79,23.62 69.79,29.76 72.99,32.09 76.38,32.09 | VLHKOST.3 76.38,32.09 | 76.38,32.09 78.24,33.95 v78.24,36.1 | C8.+ 33.39,83.78
  Bottom 1.016: IC1.7 48.57,41.42 C3.1
  Bottom 1.27: PROG.2 46.62,92.45 33.7,92.45 | 33.7,92.45 28.71,92.45 P1.1 | IC4.OUT 4.27,81.79 7.91,76.81 30.79,76.81 32.17,78.19 33.39,79.41 33.39,83.78 33.39,92.14 33.7,92.45
(copper drawn outside any net)
  shapes: Bottom circle x3

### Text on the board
Bottom: 096-011018 | PIHRT.COM | V1.0 | +3V

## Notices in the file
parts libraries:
Copyright (C) PaJa 2001-2014
SparkFun-Electromechanical: Licensing: Creative Commons ShareAlike 4.0 International - https://creativecommons.org/licenses/by-sa/4.0
Copyright (C) PaJa 2011-2014
